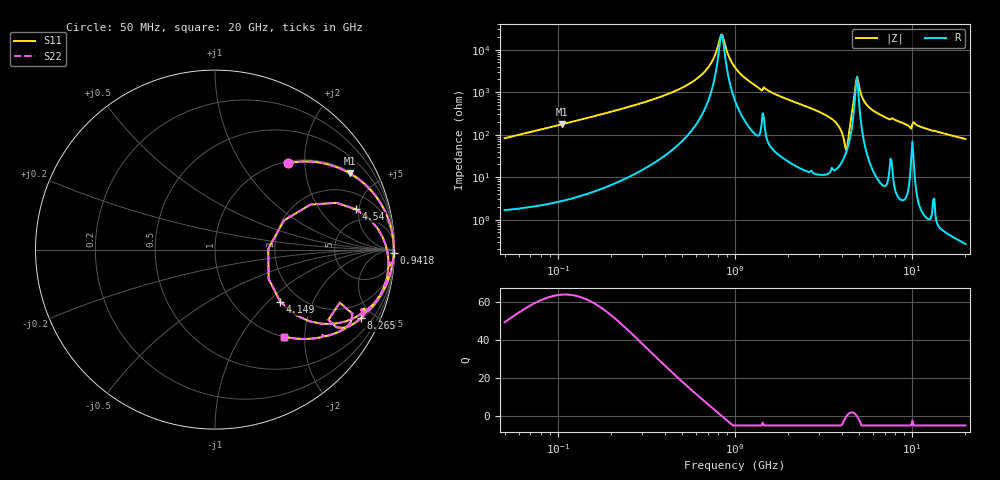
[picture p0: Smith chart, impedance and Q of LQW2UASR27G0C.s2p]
!Murata Part Number: LQW2UASR27G0C
!These Parameters are Measured in Series Mode Connection
!  o--[Z]--o
!Port1  Port2
!  o-------o
!Freq. Start=50[MHz] Stop=20[GHz], 401[Steps]
# Hz S RI R 50
!Freq.(Hz) S11(Real) S11(Imag) S21(Real) S21(Imag) S12(Real) S12(Imag) S22(Real) S22(Imag)
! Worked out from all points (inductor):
!   401 points, 50 MHz to 20 GHz, reference 50 ohm
!   read as one part in series: L = 261 nH near 51.52 MHz
!   highest Q = 63.8 at 105.7 MHz (marker M1), where L = 264 nH
!   self-resonance near 835.5 MHz
!   S11 on the Smith chart (normalised r, x): 50 MHz: 1.03, +1.64; 941.8 MHz: open; 4.149 GHz: 1.60, -1.19; 4.54 GHz: 3.45, +4.67; 8.265 GHz: 1.07, -4.20; 20 GHz: 1.01, -1.58
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5e7  0.4055 0.4809  0.5945 -0.4809  0.5945 -0.4809  0.4055 0.4809
1.057371e8  0.752 0.4241  0.248 -0.4241  0.248 -0.4241  0.752 0.4241
1.364002e8  0.8359 0.3624  0.1641 -0.3624  0.1641 -0.3624  0.8359 0.3624
3.721004e8  0.9785 0.1291  0.0215 -0.1291  0.0215 -0.1291  0.9785 0.1291
6.476653e8  0.9943 0.0383  0.00575 -0.0383  0.00575 -0.0383  0.9943 0.0383
7.411344e8  0.9954 0.0184  0.00461 -0.0184  0.00461 -0.0184  0.9954 0.0184
8.354841e8  0.9957 0.000927  0.00428 -0.000927  0.00428 -0.000927  0.9957 0.000927
9.418449e8  0.9954 -0.0167  0.00459 0.0167  0.00459 0.0167  0.9954 -0.0167
1e9  0.995 -0.0256  0.00499 0.0256  0.00499 0.0256  0.995 -0.0256
1.369645e9  0.9873 -0.0793  0.0127 0.0793  0.0127 0.0793  0.9873 -0.0793
2.728004e9  0.9363 -0.2282  0.0637 0.2282  0.0637 0.2282  0.9363 -0.2282
3.626126e9  0.8026 -0.3653  0.1974 0.3653  0.1974 0.3653  0.8026 -0.3653
3.967106e9  0.5963 -0.4134  0.4037 0.4134  0.4037 0.4134  0.5963 -0.4134
4.149438e9  0.3643 -0.2907  0.6357 0.2907  0.6357 0.2907  0.3643 -0.2907
4.275624e9  0.2964 0.00395  0.7036 -0.00395  0.7036 -0.00395  0.2964 0.00395
4.539627e9  0.7863 0.2243  0.2137 -0.2243  0.2137 -0.2243  0.7863 0.2243
4.748272e9  0.9341 0.0685  0.0659 -0.0685  0.0659 -0.0685  0.9341 0.0685
4.89267e9  0.96 -0.0109  0.04 0.0109  0.04 0.0109  0.96 -0.0109
5.598765e9  0.9465 -0.1944  0.0535 0.1944  0.0535 0.1944  0.9465 -0.1944
7.442007e9  0.8249 -0.3504  0.1751 0.3504  0.1751 0.3504  0.8249 -0.3504
8.264682e9  0.8113 -0.3828  0.1887 0.3828  0.1887 0.3828  0.8113 -0.3828
2e10  0.384 -0.4847  0.616 0.4847  0.616 0.4847  0.384 -0.4847
